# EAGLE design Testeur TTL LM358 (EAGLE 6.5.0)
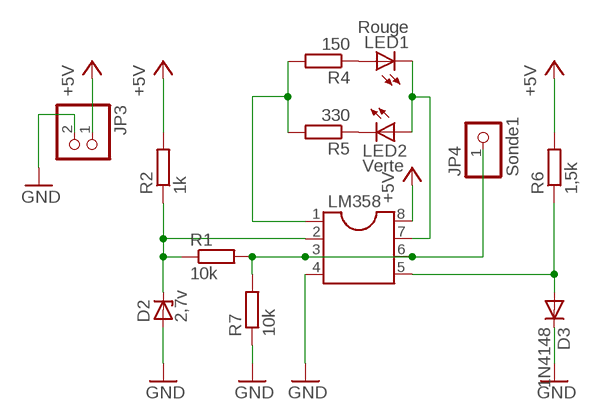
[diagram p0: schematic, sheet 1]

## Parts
D2  2,7v  BZV10  [DO34Z7]
D3  1N4148  1N4148DO35-10  [DO35-10]
JP3  PINHD-1X2  [1X02]
JP4  Sonde1  PINHD-1X1  [1X01]
LED1  Rouge  LED5MM  [LED5MM]
LED2  Verte  LED5MM  [LED5MM]
LM358  DIL8S  [SOCKET-08]
R1  10k  R-EU_0309/10  [0309/10]
R2  1k  R-EU_0309/10  [0309/10]
R4  150  R-EU_0309/10  [0309/10]
R5  330  R-EU_0309/10  [0309/10]
R6  1,5k  R-EU_0309/10  [0309/10]
R7  10k  R-EU_0309/10  [0309/10]

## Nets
+5V: JP3.1 LM358.8 R2.2 R6.2
GND: D2.A D3.C JP3.2 LM358.4 R7.1
N$1: LED1.A R4.1
N$2: JP4.1 LM358.3 LM358.6 R1.2 R7.2
N$3: D2.C LM358.2 R1.1 R2.1
N$4: LED2.K(C) R5.1
N$5: LM358.1 R4.2 R5.2
N$6: LED1.K(C) LED2.A LM358.7
N$7: D3.A LM358.5 R6.1

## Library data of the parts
D2 = diode:BZV10: Z DIODE
D3 = diode:1N4148: DIODE
JP3 = pinhead:PINHD-1X2: PIN HEADER
JP4 = pinhead:PINHD-1X1: PIN HEADER
LED1 LED2 = led:LED: LED
LM358 = ic-package:DIL8: Dual In Line / Socket
R1 R2 R4-R7 = rcl:R-EU_: RESISTOR, European symbol

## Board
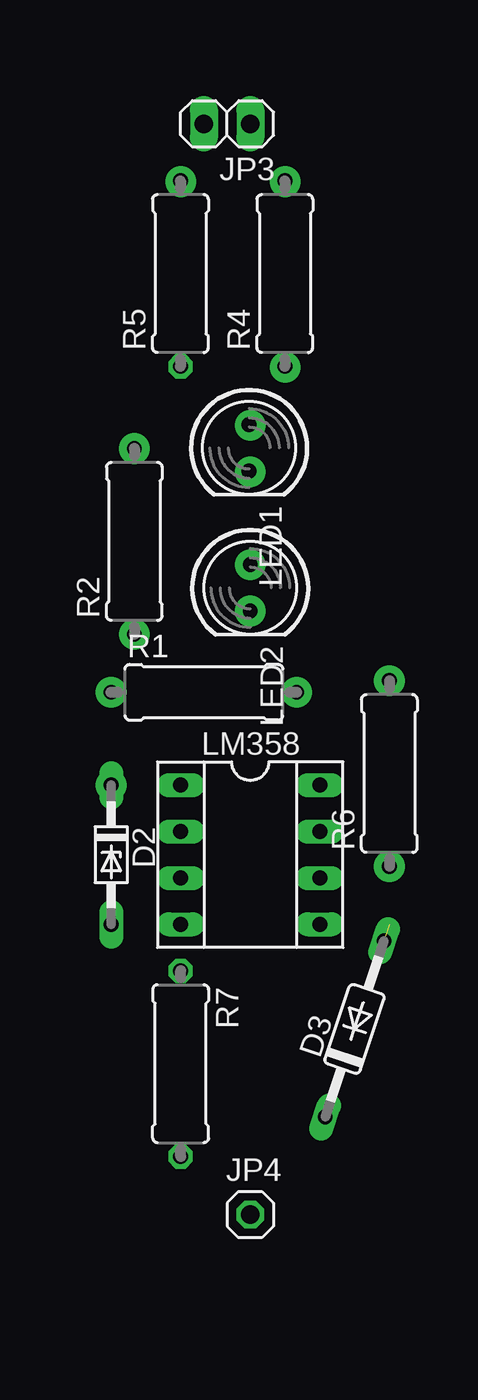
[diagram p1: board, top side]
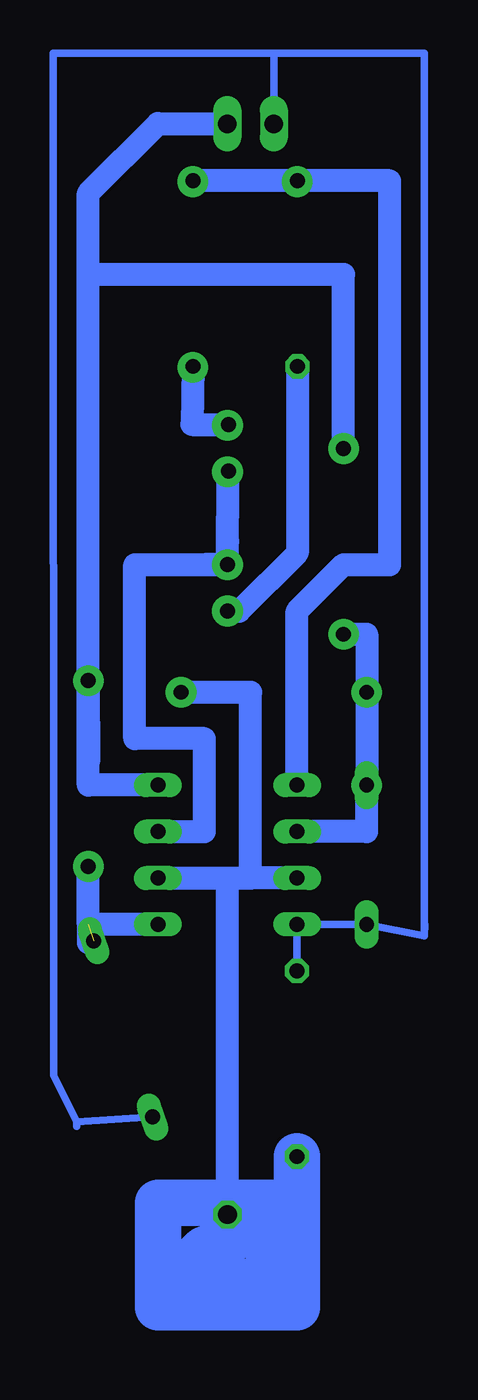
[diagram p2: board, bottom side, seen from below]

No outline drawn. Coordinates in mm, seen from the top.
Copper layers (1*16): Top 0.035mm / dielectric 1.5mm / Bottom 0.035mm
Design rules "default": minimum track width 10mil, minimum drill 24mil, track to track 8mil, track to pad 8mil, pad to pad 8mil, via to via 8mil, smd to smd 8mil, copper to edge 40mil, drill to drill 8mil, minimum pad ring 10mil, minimum via ring 8mil, stop-mask expansion 4mil, vias tented up to drill 0mil, thermal gap 10mil

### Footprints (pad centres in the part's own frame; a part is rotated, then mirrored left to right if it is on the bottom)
DO34Z7 = drill 0.813 long: A 3.81,0; C -3.81,0
DO35-10 = drill 0.813 long: A 5.08,0; C -5.08,0
1X02 = drill 1.016 long: 1 -1.27,0; 2 1.27,0
1X01 = drill 1.016 octagon: 1 0,0
LED5MM = drill 0.813 octagon: A -1.27,0; K 1.27,0
SOCKET-08 = drill 0.813 long: 1 -3.81,-3.81; 2 -1.27,-3.81; 3 1.27,-3.81; 4 3.81,-3.81; 5 3.81,3.81; 6 1.27,3.81; 7 -1.27,3.81; 8 -3.81,3.81
0309/10 = drill 0.813 octagon: 1 -5.08,0; 2 5.08,0

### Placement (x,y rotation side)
D2  13.98,20.32 270 top
D3  27.3,10.79 71.5 top
JP3  20.33,60.32 180 top
JP4  21.59,0.64 0 top
LED1  21.53,42.58 270 top
LED2  21.59,34.92 270 top
LM358  21.59,20.32 270 top
R1  19.05,29.21 0 top
R2  15.25,37.47 90 top
R4  23.48,52.12 90 top
R5  17.77,52.12 90 top
R6  29.21,24.77 90 top
R7  17.78,8.89 270 top

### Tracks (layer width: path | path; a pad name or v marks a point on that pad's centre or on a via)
+5V  (via drill 0.6 pad 1.68)
  Bottom 0.406: R6.2 29.23,25.4
  Bottom 1.27: LM358.8 29.21,24.13 v29.21,29.84 R6.2 | R6.2 29.2,25.4 | R2.2 15.25,52.06 | 15.25,52.06 15.24,52.07 | R6.2 29.21,52.07 | 15.25,52.06 29.21,52.07 | 29.21,52.07 29.21,56.52 25.4,60.33 JP3.1
GND
  Bottom 0.406: 10.8,15.88 10.8,64.18 19.05,64.18 | 19.05,64.18 31.14,64.18 31.11,8.26 29.84,5.71 | D2.A LM358.4 R7.1 | 14.23,16.25 D2.A | JP3.2 19.06,62.91 19.05,64.18 | D2.A 10.8,15.88 | 10.79,16.51 10.8,15.88 | 29.84,5.46 29.84,5.71 | D3.C 29.84,5.71
N$1
  Bottom 1.27: R4.1 23.53,43.87 LED1.A
N$2  (via drill 0.6 pad 1.68)
  Bottom 1.27: 21.61,0.64 JP4.1 21.59,19.05 | 20.32,19.05 20.32,29.21 R1.2 | LM358.6 21.59,19.05 | 21.59,19.05 20.32,19.05 | LM358.3 20.32,19.05
  Bottom 2.54: R7.2 17.78,-4.45 25.4,-4.45 25.4,1.27 18.41,1.27 19.68,-3.17 24.13,-2.54 22.86,-1.27 19.68,0 JP4.1
  other vias: 24.13,29.21
N$3  (via drill 0.6 pad 1.68)
  Bottom 1.27: R1.1 | R1.1 D2.C 13.98,21.6 13.97,21.59 LM358.2 | R2.1 13.97,32.39 13.97,32.38 R1.1
  other vias: 13.97,29.21
N$4
  Bottom 1.27: R5.1 17.77,36.84 20.95,33.66 LED2.K
N$5
  Bottom 1.27: R4.2 R5.2 12.71,57.2 12.71,36.2 15.24,36.2 17.78,33.66 LM358.1
N$6  (via drill 0.6 pad 1.68)
  Bottom 1.27: LM358.7 22.86,21.59 22.86,26.67 26.67,26.67 26.67,36.2 v21.59,36.2 22.86,36.2 LED2.A 21.59,37.47 21.59,38.73 v21.59,41.27 21.59,41.34 LED1.K
N$7  (via drill 0.6 pad 1.68)  (1 unrouted)
  Bottom 1.27: LM358.5 29.21,16.51 | 29.21,16.51 v29.21,19.68 R6.1 | 29.21,16.51 29.21,15.51
N$8  (via drill 0.6 pad 1.68)
  other vias: 15.24,32.38
N$9  (via drill 0.6 pad 1.68)
  other vias: 13.97,24.13
N$10  (via drill 0.6 pad 1.68)
  other vias: 21.59,33.66
N$11  (via drill 0.6 pad 1.68)
  other vias: 21.59,43.81
N$12  (via drill 0.6 pad 1.68)
  other vias: 23.5,46.99
N$13  (via drill 0.6 pad 1.68)
  other vias: 15.24,42.55
N$14  (via drill 0.6 pad 1.68)
  other vias: 23.5,57.15
N$15  (via drill 0.6 pad 1.68)
  other vias: 17.78,57.15

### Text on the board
Document: +5vcc | Testeur TTL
